(* Logix 5000 AddOnInstructionDefinition export AMCI_SMD34E2_Home_CCW; software revision 20.03 *)

ADD_ON_INSTRUCTION AMCI_SMD34E2_Home_CCW   (* revision 1.0, vendor AMCI *)
VAR_INPUT
   Type_0_for_standard_1_for_indexed : BOOL;
   Programmed_Speed : DINT; {required}
   Acceleration : INT; {required}
   Deceleration : INT; {required}
   Jerk : INT;
END_VAR
VAR_IN_OUT
   AMCI_SMD34E2_output_data : _000A:SMD34E2_788832CB:O:0; {required}
END_VAR
VAR
   Upper_Result_X_1000 : DINT;
   command_data_block : INT[10];
        [0]   // Command Bits MSW
        [1]   // Command Bits LSW
        [2]   // Upper Target Position
        [3]   // Lower Target Position
        [4]   // Upper Programmed Speed
        [5]   // Lower Programmed Speed
END_VAR

ROUTINE Logic   (* ladder *)
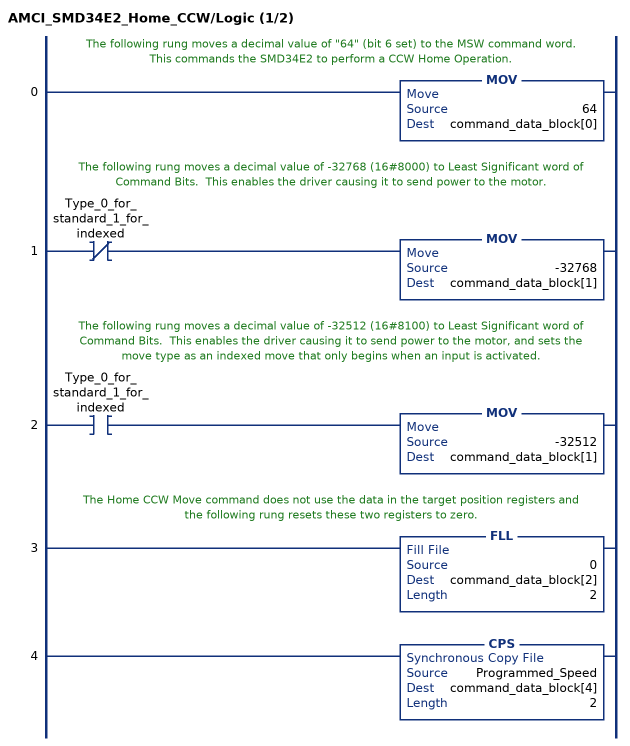
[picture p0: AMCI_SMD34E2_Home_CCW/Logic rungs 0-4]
   // The following rung moves a decimal value of "64" (bit 6 set) to the MSW command word.  This commands the SMD34E2 to perform a CCW Home Operation.
   0: MOV(64,command_data_block[0]);
   // The following rung moves a decimal value of -32768 (16#8000) to Least Significant word of Command Bits.  This enables the driver causing it to send power to the motor.
   1: XIO(Type_0_for_standard_1_for_indexed)MOV(-32768,command_data_block[1]);
   // The following rung moves a decimal value of -32512 (16#8100) to Least Significant word of Command Bits.  This enables the driver causing it to send power to the motor, and sets the move type as an indexed move that only begins when an input is activated.
   2: XIC(Type_0_for_standard_1_for_indexed)MOV(-32512,command_data_block[1]);
   // The Home CCW Move command does not use the data in the target position registers and the following rung resets these two registers to zero.
   3: FLL(0,command_data_block[2],2);
   4: CPS(Programmed_Speed,command_data_block[4],2);
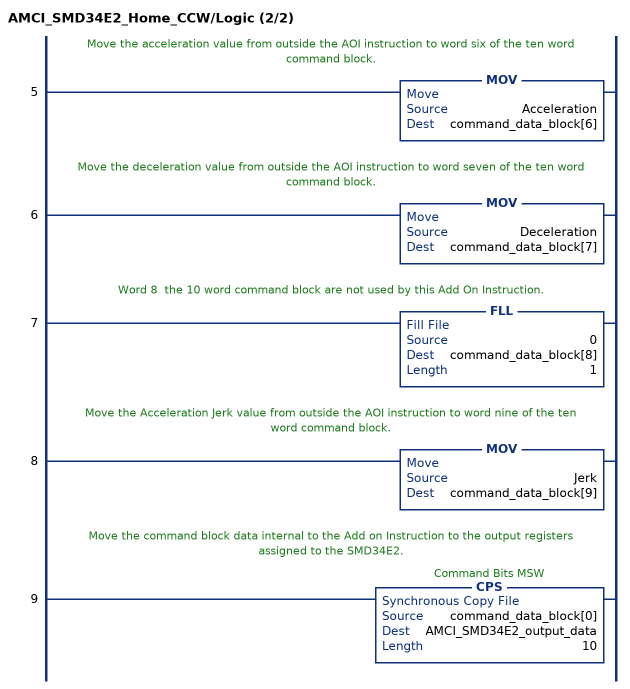
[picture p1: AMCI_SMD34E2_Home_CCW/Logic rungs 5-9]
   // Move the acceleration value from outside the AOI instruction to word six of the ten word command block.
   5: MOV(Acceleration,command_data_block[6]);
   // Move the deceleration value from outside the AOI instruction to word seven of the ten word command block.
   6: MOV(Deceleration,command_data_block[7]);
   // Word 8  the 10 word command block are not used by this Add On Instruction.
   7: FLL(0,command_data_block[8],1);
   // Move the Acceleration Jerk value from outside the AOI instruction to word nine of the ten word command block.
   8: MOV(Jerk,command_data_block[9]);
   // Move the command block data internal to the Add on Instruction to the output registers assigned to the SMD34E2.
   9: CPS(command_data_block[0],AMCI_SMD34E2_output_data,10);
END_ROUTINE
END_ADD_ON_INSTRUCTION
